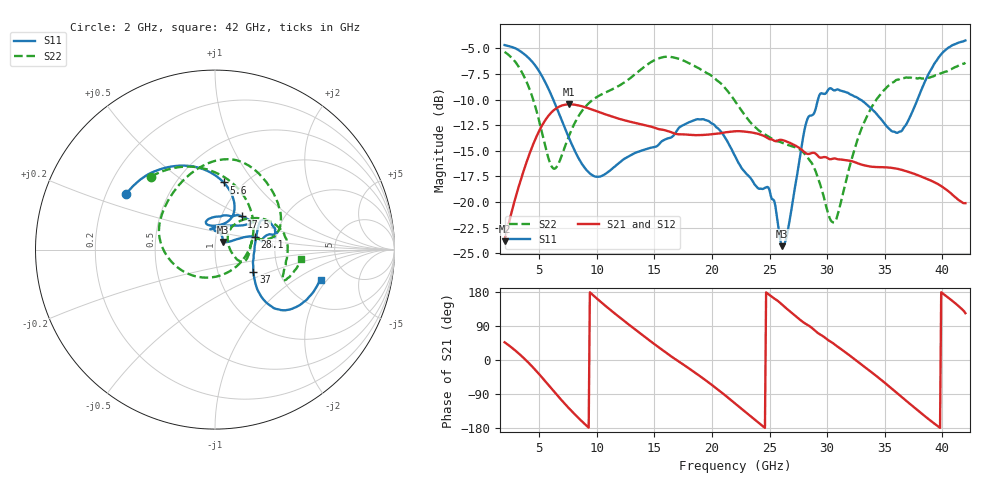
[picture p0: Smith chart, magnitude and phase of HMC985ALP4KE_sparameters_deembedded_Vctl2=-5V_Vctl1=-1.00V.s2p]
!s2p File: Measurements: S11, S21, S12, S22
# GHz S dB R 50.0
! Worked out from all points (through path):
!   401 points, 2 GHz to 42 GHz, reference 50 ohm
!   highest |S21| = -10.46 dB at 7.6 GHz (marker M1); lowest = -23.8 dB at 2 GHz (marker M2)
!   lowest |S11| = -24.3 dB at 26.1 GHz (marker M3), VSWR 1.13, Z = 54.3 + j4.66 ohm
!   |S11| at or under -10 dB: 6.223 GHz to 29.2 GHz (22.98 GHz wide, 130 % of centre); 32.87 GHz to 37.84 GHz (4.967 GHz wide, 14 % of centre)
!   |S22| runs from -22.0 to -5.3 dB; largest |S21 - S12| = 0.0003
!   S11 on the Smith chart (normalised r, x): 2 GHz: 0.28, +0.27; 5.6 GHz: 0.82, +0.72; 17.5 GHz: 1.24, +0.49; 28.1 GHz: 1.55, +0.23; 37 GHz: 1.48, -0.39; 42 GHz: 3.16, -1.74
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2  -4.68 147.7  -23.84 46.8  -23.85 46.8  -5.34 131.3
3.6  -5.47 121.1  -17.14 6.9  -17.15 6.9  -7.54 86.5
4.7  -6.74 100.2  -13.78 -27.3  -13.79 -27.3  -10.82 44.7
5.6  -8.47 82.6  -11.90 -58.6  -11.90 -58.6  -14.88 -6.5
6.4  -10.48 70.0  -10.92 -87.1  -10.93 -87.1  -16.72 -72.1
7.6  -13.78 62.4  -10.46 -127.8  -10.47 -127.8  -13.51 -143.9
8.7  -16.26 70.5  -10.65 -161.6  -10.65 -161.5  -11.14 -175.7
12  -16.13 108.8  -11.90 112.2  -11.90 112.2  -8.61 137.0
15.4  -14.37 78.8  -12.89 33.1  -12.89 33.1  -5.97 85.7
17.5  -12.50 51.2  -13.40 -11.5  -13.41 -11.5  -6.18 60.9
19.8  -12.17 36.3  -13.40 -61.4  -13.41 -61.4  -7.55 29.6
22  -15.51 53.0  -13.09 -114.5  -13.10 -114.5  -10.15 11.4
24.9  -18.58 97.4  -13.81 173.7  -13.82 173.7  -13.61 11.4
26.1  -24.31 44.6  -13.95 145.8  -13.96 145.8  -14.22 -1.6
28.1  -12.61 17.5  -15.19 96.1  -15.20 96.2  -15.39 -23.4
28.7  -11.53 10.1  -15.21 84.1  -15.21 84.1  -16.26 -25.0
30.6  -9.11 16.7  -15.74 42.2  -15.75 42.2  -21.99 20.3
33  -10.07 31.8  -16.36 -12.5  -16.36 -12.5  -12.78 46.6
35.4  -12.86 9.5  -16.64 -70.2  -16.65 -70.2  -8.59 20.2
37  -12.14 -30.3  -17.04 -111.1  -17.04 -111.0  -7.86 1.4
39.6  -6.02 -42.4  -18.23 -174.5  -18.24 -174.5  -7.59 -23.9
42  -4.23 -16.2  -20.11 123.6  -20.12 123.6  -6.39 -6.1
